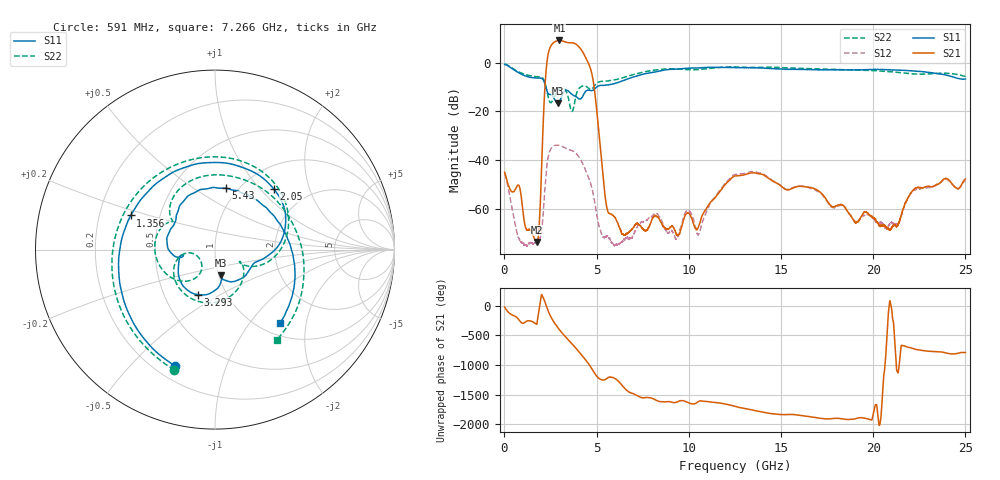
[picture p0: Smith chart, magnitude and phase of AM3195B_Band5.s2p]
!Agilent Technologies,E8364B,MY43040894,A.07.50.67
!Agilent E8364B: A.07.50.67
!Date: Wednesday, July 07, 2021 13:18:26
!Correction: S11(Full 2 Port(1,2))
!S21(Full 2 Port(1,2))
!S12(Full 2 Port(1,2))
!S22(Full 2 Port(1,2))
!S2P File: Measurements: S11, S21, S12, S22:
# Hz S  dB  R 50
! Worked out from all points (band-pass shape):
!   8001 points, 10 MHz to 25 GHz, reference 50 ohm
!   highest |S21| = 9.16 dB at 2.981 GHz (marker M1); lowest = -73.6 dB at 1.781 GHz (marker M2)
!   |S21| within 3 dB of the highest: 2.471 GHz to 4.088 GHz (1.617 GHz wide, 49.3 % of centre)
!   lowest |S11| = -16.7 dB at 2.893 GHz (marker M3), VSWR 1.34, Z = 51 - j15 ohm
!   |S11| at or under -10 dB: 2.244 GHz to 4.992 GHz (2.748 GHz wide, 76 % of centre)
!   |S22| runs from -20.0 to -0.4 dB; largest |S21 - S12| = 2.9
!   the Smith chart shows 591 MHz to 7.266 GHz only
!   S11 on the Smith chart (normalised r, x): 591 MHz: 0.28, -0.68; 1.356 GHz: 0.34, +0.17; 2.05 GHz: 1.38, +1.19; 3.293 GHz: 0.74, -0.40; 5.43 GHz: 0.88, +0.69; 7.266 GHz: 1.23, -1.43
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1e7  -0.69 -10.0  -44.96 -20.4  -45.50 -39.2  -0.45 -10.8
5.910175e8  -3.29 -109.0  -52.05 -176.7  -66.55 -134.4  -3.01 -108.7
1.356336e9  -5.91 157.9  -68.44 108.4  -74.20 150.0  -5.24 159.4
1.781166e9  -6.23 101.0  -73.61 102.4  -72.57 28.9  -5.71 102.8
2.049809e9  -6.55 45.7  -35.65 169.4  -66.88 -7.3  -6.10 47.4
2.399669e9  -12.86 -20.8  4.51 -104.0  -37.73 88.1  -14.83 -28.1
2.546485e9  -13.07 -43.3  7.24 159.6  -35.06 -6.9  -16.28 -25.5
2.70892e9  -14.90 -71.9  8.49 75.1  -34.02 -89.5  -13.82 -37.9
2.893221e9  -16.66 -77.8  9.09 -6.2  -33.77 -169.2  -11.36 -69.7
2.980686e9  -15.96 -76.9  9.16 -41.6  -33.87 156.2  -10.72 -86.0
3.293061e9  -11.43 -110.5  8.56 -155.6  -34.97 44.6  -11.09 -143.3
3.639798e9  -12.84 -153.5  8.20 89.5  -35.98 -66.4  -19.89 -153.9
3.886574e9  -13.90 -167.9  7.60 1.4  -37.20 -150.5  -13.30 -128.0
4.177082e9  -14.53 -167.4  5.26 -106.9  -40.32 106.9  -9.73 -168.1
4.53319e9  -11.20 164.4  0.18 114.4  -46.54 -25.3  -10.28 151.3
5.429706e9  -9.17 79.8  -52.67 -170.2  -71.69 -141.7  -7.57 78.3
7.266471e9  -5.23 -48.2  -66.21 -88.6  -66.55 -70.7  -4.30 -55.6
8.341041e9  -3.53 -93.6  -63.56 -171.4  -62.50 176.5  -2.84 -105.8
1.2505e10  -1.97 142.2  -46.46 99.3  -45.85 100.8  -1.71 128.6
1.667208e10  -2.83 18.3  -51.35 -79.3  -51.76 -82.1  -2.44 2.8
2.083604e10  -2.91 -71.2  -68.42 -76.5  -66.70 -117.2  -3.59 -82.4
2.5e10  -6.69 -116.1  -47.73 -69.3  -48.42 -60.8  -5.57 -124.5
